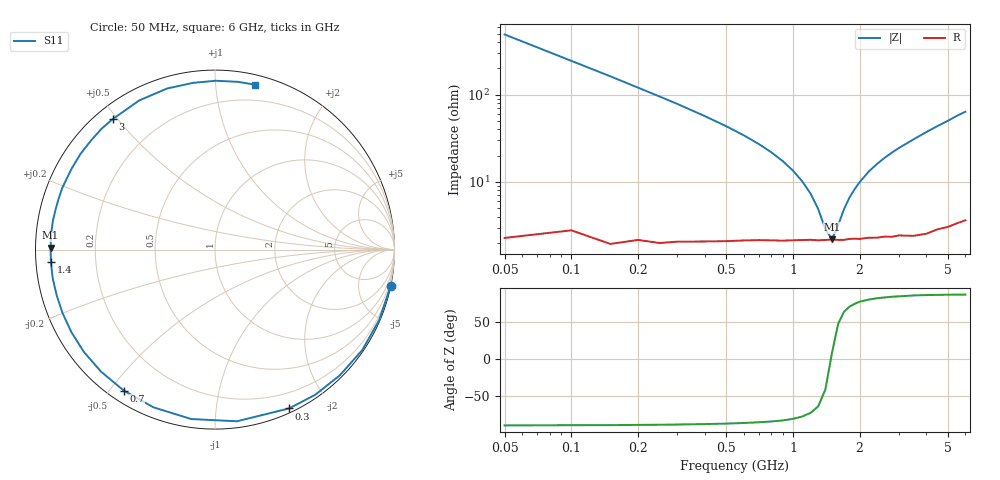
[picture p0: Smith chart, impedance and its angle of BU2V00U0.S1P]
! Infineon Technologies  Discrete & RF Semiconductors
! BB 833
! Si Tuning Diode in SOD323
! VR = 2 V
! S-Parameters:  June  1999
# GHz  S  MA  R  50
!  f  S11
! GHz  MAG  ANG
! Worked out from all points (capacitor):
!   34 points, 50 MHz to 6 GHz, reference 50 ohm
!   read as one part to ground: C = 6.51 pF near 50 MHz
!   lowest |Z| = 2.21 ohm at 1.5 GHz (marker M1)
!   series resonance near 1.486 GHz, so ESL is about 1.8 nH
!   S11 on the Smith chart (normalised r, x): 50 MHz: 0.05, -9.76; 300 MHz: 0.04, -1.57; 700 MHz: 0.04, -0.54; 1.4 GHz: 0.04, -0.04; 3 GHz: 0.05, +0.49; 6 GHz: 0.07, +1.27
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0.05  0.999 -11.7
0.1  0.9955 -23.2
0.15  0.9932 -34.3
0.2  0.9873 -45.2
0.25  0.9829 -55.4
0.3  0.9764 -65.0
0.4  0.9643 -82.7
0.5  0.9532 -98.0
0.6  0.9433 -111.3
0.7  0.9355 -122.9
0.8  0.9303 -133.0
0.9  0.9266 -142.0
1  0.9228 -150.1
1.1  0.9201 -157.4
1.3  0.9182 -169.9
1.4  0.917 -175.6
1.5  0.916 179.3
1.6  0.9169 174.6
1.8  0.9159 165.7
2  0.9176 158.0
2.4  0.9198 144.5
2.8  0.9236 133.2
3  0.924 128.1
3.5  0.9322 116.9
4  0.9363 106.6
5  0.9408 89.8
5.5  0.9433 82.3
6  0.9459 76.2
